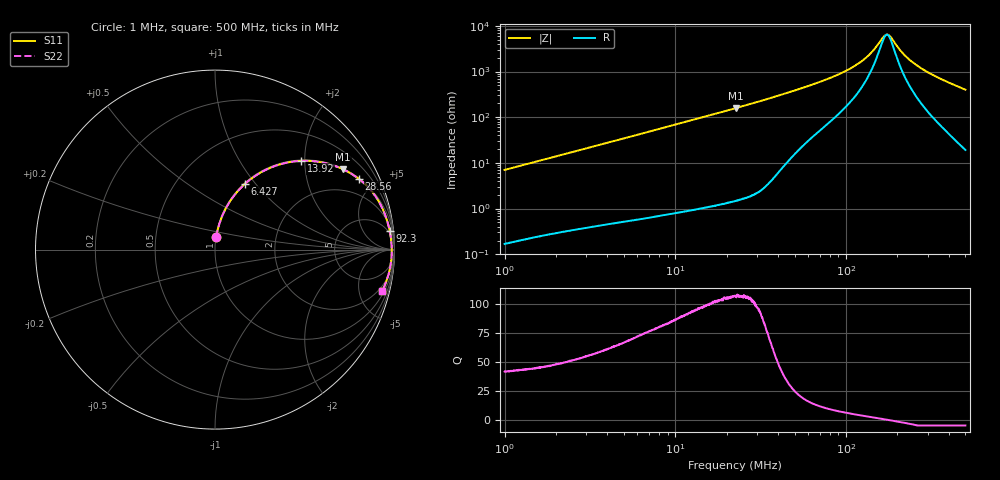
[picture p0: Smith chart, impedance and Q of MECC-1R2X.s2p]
!s-Parameter Generated by FASTRON Sdn. Bhd.
!FASTRON P/N : MECC-1R2X
!Keysight Technologies,E4991B,MY54100416,A.01.15
!Date: Mon Mar 16 14:43:52 2026
!Version  : Rev00 Mon Mar 16 14:43:52 2026
!Data & Calibration Information:
!PortZ  Port1:50+j0  Port2:50+j0
!When reading, reference impedance value at option line is always used.
! Remarks : This data is being provided solely for informational purposes.
!Freq	S11	S21	S12	S22
# Hz S dB R 50
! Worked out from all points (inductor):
!   1601 points, 1 MHz to 500 MHz, reference 50 ohm
!   read as one part in series: L = 1.11 uH near 1.032 MHz
!   highest Q = 107 at 22.71 MHz (marker M1), where L = 1.11 uH
!   self-resonance near 173.6 MHz
!   S11 on the Smith chart (normalised r, x): 1 MHz: 1.00, +0.14; 6.427 MHz: 1.01, +0.89; 13.92 MHz: 1.02, +1.92; 28.56 MHz: 1.04, +4.06; 92.3 MHz: 4, +18; 500 MHz: 1.38, -8.02
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1000000  -23.10 84.6  -0.04 -4.0  -0.04 -4.0  -23.10 84.6
2820919  -14.37 77.9  -0.19 -11.0  -0.19 -11.0  -14.37 77.9
4409396  -10.76 72.3  -0.42 -16.8  -0.42 -16.8  -10.76 72.3
6426939  -7.90 65.5  -0.82 -23.7  -0.82 -23.7  -7.90 65.5
7957584  -6.41 60.7  -1.19 -28.5  -1.19 -28.5  -6.41 60.7
1.392158e7  -3.23 45.8  -2.89 -43.6  -2.89 -43.6  -3.23 45.8
2.236068e7  -1.53 32.4  -5.41 -57.0  -5.41 -57.0  -1.53 32.4
2.27108e7  -1.48 32.0  -5.51 -57.4  -5.51 -57.4  -1.48 32.0
2.855992e7  -0.98 26.1  -7.12 -63.3  -7.12 -63.3  -0.98 26.1
4.114541e7  -0.50 17.9  -10.22 -70.8  -10.22 -70.8  -0.50 17.9
6.307767e7  -0.27 10.8  -14.51 -75.2  -14.51 -75.2  -0.27 10.8
9.229699e7  -0.19 6.2  -19.27 -75.7  -19.27 -75.7  -0.19 6.2
1.094988e8  -0.16 4.4  -22.12 -74.1  -22.12 -74.1  -0.16 4.4
1.254438e8  -0.15 3.1  -25.08 -70.7  -25.08 -70.7  -0.15 3.1
1.431536e8  -0.14 1.8  -29.07 -62.0  -29.07 -62.0  -0.14 1.8
1.672155e8  -0.13 0.3  -35.67 -21.4  -35.67 -21.4  -0.13 0.3
1.72493e8  -0.13 0.1  -36.31 -3.8  -36.31 -3.8  -0.13 0.1
1.77937e8  -0.13 -0.2  -36.10 14.9  -36.10 14.9  -0.13 -0.2
2.169182e8  -0.14 -2.2  -27.81 66.4  -27.81 66.4  -0.14 -2.2
2.603623e8  -0.15 -4.1  -22.79 74.5  -22.79 74.5  -0.15 -4.1
3.443751e8  -0.19 -7.5  -17.62 76.6  -17.62 76.6  -0.19 -7.5
5e8  -0.36 -13.8  -12.43 73.5  -12.43 73.5  -0.36 -13.8
